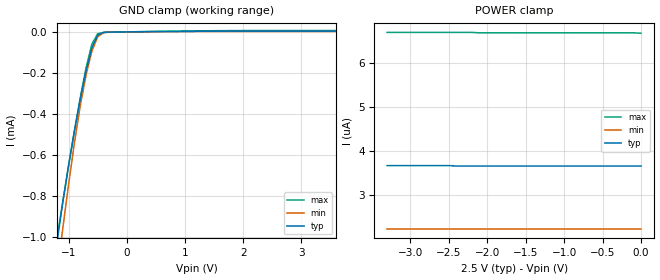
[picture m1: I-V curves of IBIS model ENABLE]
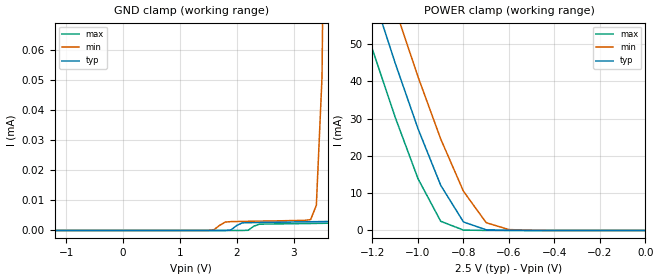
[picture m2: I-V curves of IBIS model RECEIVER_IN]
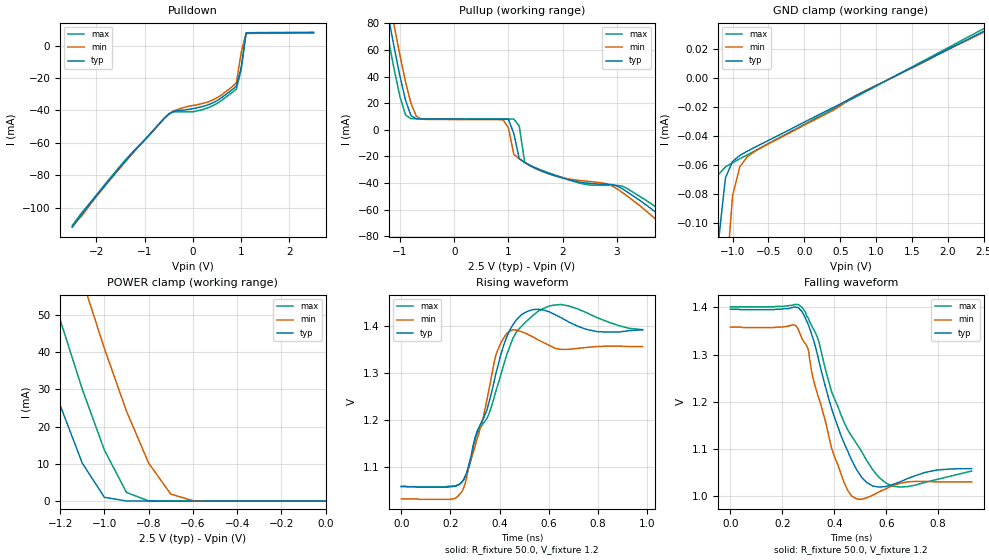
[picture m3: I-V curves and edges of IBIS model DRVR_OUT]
|   Texas Instruments Incorporated
|   Data Transmissions Products
|   IBIS Model for SN65LVDS20
|   8DRF  Small-Outline No-Lead Package
[IBIS Ver]   3.2
[Comment char]   |_char
[File name]   lvds20_2p5v.ibs
[File Rev]   1.1
[Date]   11Jun04
[Source]   File originated at Texas Instruments Incorporated.
   Data Transmission Products Group.
[Notes]
[Disclaimer]
(C) Copyright Texas Instruments Incorporated 2004
   All rights reserved
  Texas Instruments Incorporated hereby grants the user of this IBIS
model a non-exclusive, nontransferable license to use this IBIS model
under the following terms.  Before using this IBIS model, the user
should read this license.  If the user does not accept these terms,
the IBIS model should be returned to Texas Instruments within 30 days.
  The user is granted this license only to use the IBIS model and
is not granted rights to sell, load, rent, lease or license the IBIS
model in whole or in part, or in modified form to anyone other than
user.  User may modify the IBIS model to suit its specific applications
but rights to derivative works and such modifications shall belong to
Texas Instruments.
  This IBIS model is provided on an "AS IS" basis and Texas Instruments
makes absolutely no warranty with respect to the information contained
herein.  TEXAS INSTRUMENTS DISCLAIMS AND CUSTOMER WAIVES ALL WARRANTIES,
EXPRESS OR IMPLIED, INCLUDING WARRANTIES OF MERCHANTABILITY OR FITNESS
FOR A PARTICULAR PURPOSE. The entire risk as to quality and performance
is with the Customer. ACCORDINGLY, IN NO EVENT SHALL THE COMPANY BE LIABLE
FOR ANY DAMAGES, WHETHER IN CONTRACT OR TORT,INCLUDING ANY LOST PROFITS
OR OTHER INCIDENTAL, CONSEQUENTIAL, EXEMPLARY, OR PUNITIVE DAMAGES ARISING
OUT OF THE USE OR APPLICATION OF THE IBIS model provided in this package.
Further, Texas Instruments reserves the right to discontinue or make changes
without notice to any product herein to improve reliability, function, or
design. Texas Instruments does not convey any license under patent rights
or any other intellectual property rights, including those of third parties.
Contact Texas Instruments at ATTN:DATA TRANSMISSIONS
[Copyright]   Copyright 2004, Texas Instruments, All Rights Reserved
[Component]   LVDS20DRF
[Manufacturer]  Texas Instruments Incorporated
[Package]
|   typ   min   max
R_pkg   0.189   0.176   0.203
L_pkg   0.802nH   0.759nH   0.850nH
C_pkg   0.053pF   0.046pF   0.067pF
[Pin]   signal_name   model_name   R_pin   L_pin   C_pin
1   NC   NC   0.194   0.817n   0.054p
2   A   RECEIVER_IN   0.193   0.814n   0.054p
3   B   RECEIVER_IN   0.187   0.793n   0.052p
4   VBB   POWER   0.194   0.821n   0.054p
5   EN/   ENABLE   0.176   0.759n   0.046p
6   Z   DRVR_OUT   0.188   0.799n   0.051p
7   Y   DRVR_OUT   0.181   0.772n   0.050p
8   VCC   POWER   0.187   0.791n   0.052p
9   GND   GND   0.203   0.850n   0.067p
[Diff_pin]   inv_pin   vdiff   tdelay_typ   tdelay_min   tdelay_max
| The 'A/Y' pin is Diff_pin and the 'B/Z' pin is the inv_pin
2   3   0.100   0 0 0
7   6   0.000   0 0 0
| Models and submodels in the file (3): ENABLE (Input), RECEIVER_IN (Input), DRVR_OUT (3-state)
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|   Enable Input Model
[Model]   ENABLE
Model_type   Input
|Signals   /E
Vinh = 2.0
Vinl = 0.8
C_comp   3.3pF   3.28pF   3.38pF
|   typ   min   max
[Temperature Range]   25   -40   85
[Voltage range]   2.5V   2.375V   2.625V
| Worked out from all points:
|   GND clamp passes 1 mA (typ) near -1.18 V on its own axis
[GND_clamp]
|Voltage I(typ)   I(min)   I(max)
-3.6V     -6.81mA    -7.03mA    -6.59mA
-1.2V     -1.03mA    -1.18mA    -1.01mA
-1.1V     -834uA     -961uA     -829uA
-1V       -652uA     -745uA     -654uA
-900mV    -485uA     -543uA     -484uA
-800mV    -330uA     -362uA     -323uA
-700mV    -191uA     -211uA     -176uA
-600mV    -78.2uA    -93.9uA    -60.7uA
-500mV    -15.7uA    -24.3uA    -8.94uA
-400mV    -2.37uA    -3.64uA    -2.58uA
-300mV    -1.1uA     -901nA     -1.79uA
3.6V      3.66uA     2.24uA     6.67uA
[Power_clamp]
| Note that the[POWER_clamp]voltage table is referenced to Vcc
| and is calculated using Vtable=Vcc - Vmeasured.
|Voltage I(typ)   I(min)   I(max)
-3.3V     3.67uA     2.24uA     6.69uA
-2.5V     3.67uA     2.24uA     6.69uA
-2.4V     3.66uA     2.24uA     6.69uA
-2.2V     3.66uA     2.24uA     6.69uA
-2.1V     3.66uA     2.24uA     6.68uA
-100mV    3.66uA     2.24uA     6.68uA
0V        3.66uA     2.24uA     6.67uA
|   Receiver Input Model
[Model]   RECEIVER_IN
Model_type   Input
|Signals   A, B
Vinh = 2.2
Vinl = 1.8
|   typ   min   max
C_comp   1.0pF   0.98pF   1.10pF
|   typ   min   max
[Temperature Range]   25   -40   85
[Voltage range]   2.5V   2.375V   2.625V
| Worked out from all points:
|   POWER clamp passes 1 mA (typ) near -0.74 V on its own axis
[GND_clamp]
|Voltage I(typ)   I(min)   I(max)
-3.6V     -93.5pA    -92.3pA    -96.3pA
1.5V      -4.04pA    13.2nA     -8.24pA
1.6V      125fA      270nA      -6.57pA
1.8V      4.55nA     2.8uA      -3.22pA
1.9V      186nA      2.94uA     -1.41pA
2.1V      2.52uA     3.01uA     483pA
2.2V      2.58uA     3.04uA     63.6nA
2.4V      2.64uA     3.1uA      2.1uA
3.3V      2.9uA      3.61uA     2.32uA
3.4V      2.93uA     8.35uA     2.35uA
3.5V      2.96uA     51uA       2.37uA
3.6V      2.99uA     240uA      2.4uA
[Power_clamp]
| Note that the[POWER_clamp]voltage table is referenced to Vcc
| and is calculated using Vtable=Vcc - Vmeasured.
|Voltage   I(typ)   I(min)   I(max)
-3.3V     557mA      575mA      539mA
-1.3V     83.2mA     98.5mA     67.8mA
-1.2V     63.6mA     78.6mA     48.5mA
-1.1V     44.8mA     59.4mA     30.3mA
-1V       27.3mA     41.2mA     13.9mA
-900mV    12.1mA     24.5mA     2.46mA
-800mV    2.28mA     10.5mA     111uA
-700mV    181uA      2.08mA     10.4uA
-600mV    29.5uA     240uA      2.64uA
0V        2.9uA      3.29uA     2.4uA
|   Driver Output Model
[Model]   DRVR_OUT
Model_type   3-state
| Signals   Y, Z
Vmeas = 1.2V   |Reference voltage for timing measurements
Cref = 1pF   |Timing specification test load capacitance value
Rref = 50   |Note: 50 Ohm load; single ended configuration
Vref = 1.20V   |Timing specification test load voltage
|Note: 50 Ohm load; single ended configuration
| variable   typ   min   max
C_comp   1.38pF   1.34pF   1.41pF
|   typ   min   max
[Temperature Range]   25.0   -40.0   85.0
[Voltage range]   2.5V   2.375V   2.625V
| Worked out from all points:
|   slope of the pulldown table from 0 to 0.375 V, typ, clamps not added: 121 ohm
|   slope of the pullup table from 0 to 0.375 V, typ, clamps not added: 6.52 kohm
|   GND clamp passes 1 mA (typ) near -1.45 V on its own axis
|   POWER clamp passes 1 mA (typ) near -0.99 V on its own axis
|   rising waveform, R_fixture 50.0, V_fixture 1.2: 20-80 % time 114ps typ, 93.9ps min, 133ps max; typ from 1.06 V to 1.39 V
|   falling waveform, R_fixture 50.0, V_fixture 1.2: 20-80 % time 106ps typ, 88.6ps min, 134ps max; typ from 1.4 V to 1.06 V
[Pulldown]
|Voltage I(typ)   I(min)   I(max)
-2.5V     -112mA     -112mA     -111mA
-2.2V     -100mA     -101mA     -99.5mA
-1.5V     -74.8mA    -75.2mA    -74mA
-500mV    -42.2mA    -42.3mA    -42.2mA
-300mV    -40mA      -39.2mA    -40.9mA
0V        -38.9mA    -37mA      -40.9mA
300mV     -36.7mA    -34.9mA    -38.5mA
600mV     -32mA      -30.3mA    -33.7mA
900mV     -25.1mA    -23mA      -26.9mA
1V        -13.6mA    -4.2mA     -14.9mA
1.1V      7.49mA     7.42mA     7.79mA
2.5V      8.01mA     7.71mA     8.17mA
[Pullup]
|Voltage   I(typ)   I(min)   I(max)
| Note that the[Pullup]voltage table is referenced to Vcc
| and is calculated using Vtable=Vcc - Vmeasured.
-2.5V     412mA      430mA      395mA
-1.3V     104mA      121mA      87.1mA
-1.2V     81.8mA     98.4mA     64.8mA
-1.1V     60.2mA     76.5mA     43.7mA
-800mV    10.8mA     20.1mA     8.34mA
900mV     7.87mA     7.54mA     8.06mA
1.1V      -2.86mA    -18.5mA    8.03mA
1.2V      -21.7mA    -21.8mA    2.76mA
1.4V      -27mA      -27mA      -26.8mA
2.9V      -41.1mA    -42mA      -41.8mA
4V        -71.6mA    -77.5mA    -66.5mA
5V        -110mA     -117mA     -103mA
[GND_clamp]
|Voltage   I(typ)   I(min)   I(max)
-2.5V     -16.7mA    -20.1mA    -13.7mA
-1.4V     -675uA     -1.36mA    -215uA
-1.3V     -276uA     -722uA     -90.9uA
-1.2V     -114uA     -329uA     -66.4uA
-1.1V     -68.6uA    -145uA     -61uA
-1V       -57.2uA    -80.8uA    -58.1uA
-900mV    -53.1uA    -61uA      -55.4uA
-800mV    -50.3uA    -54.2uA    -52.8uA
-500mV    -42.7uA    -45.1uA    -44.9uA
400mV     -20.1uA    -22uA      -21.1uA
700mV     -12.5uA    -12.2uA    -13.2uA
2.5V      32.5uA     31.8uA     34.3uA
[Power_clamp]
| Note that the[POWER_clamp]voltage table is referenced to Vcc
| and is calculated using Vtable=Vcc - Vmeasured.
|Voltage   I(typ)   I(min)   I(max)
-2.5V     333mA      410mA      367mA
-1.4V     63.6mA     122mA      90.4mA
-1.3V     43.8mA     100mA      68.8mA
-1.2V     25.7mA     79.2mA     48.6mA
-1.1V     10.2mA     59.3mA     30mA
-1V       1.06mA     40.9mA     13.7mA
-900mV    68.6uA     24.1mA     2.34mA
-800mV    55.5uA     10.2mA     94.4uA
-700mV    52.8uA     1.9mA      56.3uA
-600mV    50.1uA     153uA      53.4uA
0V        34.3uA     28.8uA     37.6uA
[Ramp]
|   typ   min   max
dV/dt_r   0.202/112ps   0.196/98ps   0.201/151ps
dV/dt_f   0.203/100ps   0.197/90ps   0.209/133ps
R_load = 50ohm |Note: The measurement is on a single-ended configuration
|   with 100ohm line-to-line.
[Rising Waveform]
R_fixture = 50.0
V_fixture = 1.2
C_fixture = 0p
L_fixture = 0n
|   V(typ)  V(min)  V(max)
0s        1.057V     1.031V     1.058V
243ps     1.065V     1.044V     1.065V
306ps     1.172V     1.156V     1.168V
334ps     1.203V     1.208V     1.193V
384ps     1.298V     1.338V     1.261V
441ps     1.392V     1.39V      1.357V
511ps     1.432V     1.384V     1.412V
626ps     1.425V     1.353V     1.446V
795ps     1.389V     1.357V     1.419V
981ps     1.393V     1.357V     1.393V
[Falling Waveform]
R_fixture = 50.0
V_fixture = 1.2
C_fixture = 0p
L_fixture = 0n
|   V(typ)  V(min)  V(max)
0s        1.396V     1.358V     1.401V
254ps     1.4V       1.36V      1.406V
298ps     1.366V     1.314V     1.379V
334ps     1.303V     1.219V     1.338V
390ps     1.185V     1.101V     1.221V
467ps     1.076V     1V         1.127V
524ps     1.029V     996mV      1.076V
623ps     1.024V     1.022V     1.021V
749ps     1.05V      1.031V     1.029V
929ps     1.058V     1.03V      1.053V
